| NXP Semiconductors
| Logic Products Group
| IBIS model of NX3DV3899
| DUAL DOUBLE-POLE DOUBLE-THROW ANALOG SWITCH
|[Packages]:
|[Package1]: HXQFN16U (HR) 16-pins package
|[Package2]: XQFN16 (GU) 16-pins Package
[IBIS Ver]   3.2
[File Name]   nx3dv3899.ibs
[File Rev]   1.0
[Date]   17-Jun-2011
[Source]   File created from simulations by LPG
   NXP Semiconductors Nijmegen
[Notes]   V1.0   Ibis model.
   Revision History
   Version Date   Author/ Description
   Editor
   1.0   Juny  2011   RRV   Initial Model
   Remarks: - The Power Clamp curves have been omitted from the input
   since there is no power clamp diode.
   - IBISCHK 5.0.1 used
   - Following notes/warnings are caused by normal switch behaviour:
   'Series_MOSFET has Decreasing Current'
   'Series_MOSFET data is non-monotonic'
[Disclaimer]
   NXP Semiconductors warrants and represents that the IBIS model
   identified herein is owned by NXP Semiconductors (NXP). The
   model provided is not warranted as fully representing all of the
   operating characteristics and specifications of the semiconductor
   products to which the model relates.  Moreover, unless there is a
   signed, written agreement to the contrary, this IBIS model is
   furnished on an "as is" basis without support or warranty of any
   kind, either expressed or implied, regarding the use thereof, and
   NXP specifically disclaims all implied warranties of
   merchantability and fitness of the model for any purpose.
   NXP does not assume any liability arising out of the application
   or use of this IBIS model including infringement of patents and
   copyrights, nor does NXP convey any license under its patents and
   copyrights or the rights of others.
   NXP provides IBIS models as a service to our customers. You and
   your company shall not distribute, convey, sell, or give these models
   to anyone else without receiving prior written permission from
   NXP.
   NXP reserves the right to make changes without notice to these
   IBIS models to improve reliability, function, or design.
   Please be aware that your receipt and subsequent use of the IBIS
   information provided shall serve as acceptance of the terms and
   conditions of this agreement.  If you do not accept these terms,
   you should return or destroy the IBIS models and any other
   accompanying information immediately.
[Copyright]
   (C) Copyright 2011 NXP Semiconductors
   All rights reserved
|   Info for  HXQFN16U (HR) 16-pins package
[Component]   NX3DV3899_HR
[Manufacturer]   NXP Semiconductors
[Package]
|   Typ   Min   Max
R_pkg   6.915E-02   6.329E-02   7.890E-02
L_pkg   1.056E-09   9.663E-10   1.206E-09
C_pkg   1.547E-13   1.500E-13   1.640E-13
[Pin] signal_name   model_name   R_pin   L_pin   C_pin
   1   1Y0   NX3DV3899_TERM1 7.110E-02 1.086E-09 1.548E-13
   2   1S   NX3DV3899_CTRLIN 6.330E-02 9.663E-10 1.500E-13
   3   2Y1   NX3DV3899_TERM1 6.329E-02 9.663E-10 1.502E-13
   4   2Z   NX3DV3899_TERM2 7.110E-02 1.086E-09 1.550E-13
   5   2Y0   NX3DV3899_TERM1 7.889E-02 1.206E-09 1.639E-13
   6   GND   GND 6.330E-02 9.663E-10 1.500E-13
   7   3Y1   NX3DV3899_TERM1 6.330E-02 9.664E-10 1.500E-13
   8   3Z   NX3DV3899_TERM2 7.890E-02 1.206E-09 1.639E-13
   9   3Y0   NX3DV3899_TERM1 7.110E-02 1.086E-09 1.549E-13
   10   2S   NX3DV389_CTRLIN 6.330E-02 9.663E-10 1.500E-13
   11   4Y1   NX3DV3899_TERM1 6.330E-02 9.663E-10 1.500E-13
   12   4Z   NX3DV3899_TERM2 7.110E-02 1.086E-09 1.548E-13
   13   4Y0   NX3DV3899_TERM1 7.890E-02 1.206E-09 1.640E-13
   14   VCC   POWER 6.330E-02 9.663E-10 1.502E-13
   15   1Y1   NX3DV3899_TERM1 6.329E-02 9.663E-10 1.500E-13
   16   1Z   NX3DV3899_TERM2 7.889E-02 1.206E-09 1.638E-13
|   Info for  XQFN16 (GU) 16-pins Package
[Component]   NX3DV3899_GU
[Manufacturer]   NXP Semiconductors
[Package]
|   Typ   Min   Max
R_pkg   5.140E-02   3.890E-02   6.732E-02
L_pkg   6.558E-10   4.951E-10   8.595E-10
C_pkg   1.383E-13   1.222E-13   1.574E-13
[Pin] signal_name   model_name   R_pin   L_pin   C_pin
   1   1Y0   NX3DV3899_TERM1 4.876E-02 6.219E-10 1.378E-13
   2   1S   NX3DV3899_CTRLIN 4.180E-02 5.321E-10 1.297E-13
   3   2Y1   NX3DV3899_TERM1 4.031E-02 5.157E-10 1.286E-13
   4   2Z   NX3DV3899_TERM2 3.890E-02 4.951E-10 1.224E-13
   5   2Y0   NX3DV3899_TERM1 6.525E-02 8.353E-10 1.574E-13
   6   GND   GND 5.937E-02 7.574E-10 1.499E-13
   7   3Y1   NX3DV3899_TERM1 5.708E-02 7.305E-10 1.481E-13
   8   3Z   NX3DV3899_TERM2 5.905E-02 7.534E-10 1.454E-13
   9   3Y0   NX3DV3899_TERM1 5.082E-02 6.479E-10 1.359E-13
   10   2S   NX3DV389_CTRLIN 4.579E-02 5.835E-10 1.301E-13
   11   4Y1   NX3DV3899_TERM1 4.055E-02 5.163E-10 1.241E-13
   12   4Z   NX3DV3899_TERM2 6.732E-02 8.595E-10 1.550E-13
   13   4Y0   NX3DV3899_TERM1 3.894E-02 4.957E-10 1.222E-13
   14   VCC   POWER 4.994E-02 6.366E-10 1.349E-13
   15   1Y1   NX3DV3899_TERM1 5.901E-02 7.529E-10 1.454E-13
   16   1Z   NX3DV3899_TERM2 5.948E-02 7.590E-10 1.459E-13
[Series Pin Mapping]  pin_2  model_name   function_table_group
 4   5   NX3DV3899_SWITCH1   1
 4   3   NX3DV3899_SWITCH1   2
 8   9   NX3DV3899_SWITCH1   1
 8   7   NX3DV3899_SWITCH1   2
12   13   NX3DV3899_SWITCH1   1
12   11   NX3DV3899_SWITCH1   2
16   1   NX3DV3899_SWITCH1   1
16   15   NX3DV3899_SWITCH1   2
 5   4   NX3DV3899_SWITCH2   3
 3   4   NX3DV3899_SWITCH2   4
 9   8   NX3DV3899_SWITCH2   3
 7   8   NX3DV3899_SWITCH2   4
13   12   NX3DV3899_SWITCH2   3
11   12   NX3DV3899_SWITCH2   4
 1   16   NX3DV3899_SWITCH2   3
15   16   NX3DV3899_SWITCH2   4
[Series Switch Groups]
| Function Group States
On 1 /   | Z  to Y0, S=Low
On 2 /   | Z  to Y1, S=High
On 3 /   | Y0 to Z, S=Low
On 4 /   | Y1 to Z, S=High
[Model Selector]   NX3DV3899_SWITCH1
NX3DV3899_SWITCH1_33   3.3V-Vcc Series switch model
NX3DV3899_SWITCH1_25   2.5V-Vcc Series switch model
NX3DV3899_SWITCH1_18   1.8V-Vcc Series switch model
NX3DV3899_SWITCH1_15   1.5V-Vcc Series switch model
[Model Selector]   NX3DV3899_SWITCH2
NX3DV3899_SWITCH2_33   3.3V-Vcc Series switch model
NX3DV3899_SWITCH2_25   2.5V-Vcc Series switch model
NX3DV3899_SWITCH2_18   1.8V-Vcc Series switch model
NX3DV3899_SWITCH2_15   1.5V-Vcc Series switch model
[Model Selector]   NX3DV3899_TERM1
NX3DV3899_TERM1_33   3.3V-Vcc Series switch I/O model
NX3DV3899_TERM1_25   2.5V-Vcc Series switch I/O model
NX3DV3899_TERM1_18   1.8V-Vcc Series switch I/O model
NX3DV3899_TERM1_15   1.5V-Vcc Series switch I/O model
[Model Selector]   NX3DV3899_CTRLIN
NX3L_CTRLIN_33   3.3V-Vcc input model
NX3L_CTRLIN_25   2.5V-Vcc input model
NX3L_CTRLIN_18   1.8V-Vcc input model
NX3L_CTRLIN_15   1.5V-Vcc input model
[Model Selector]   NX3DV3899_TERM2
NX3DV3899_TERM2_33   3.3V-Vcc Series switch I/O model
NX3DV3899_TERM2_25   2.5V-Vcc Series switch I/O model
NX3DV3899_TERM2_18   1.8V-Vcc Series switch I/O model
NX3DV3899_TERM2_15   1.5V-Vcc Series switch I/O model
[Model Selector]   NX3DV389_CTRLIN
NX3L_CTRLIN_33   3.3V-Vcc input model
NX3L_CTRLIN_25   2.5V-Vcc input model
NX3L_CTRLIN_18   1.8V-Vcc input model
NX3L_CTRLIN_15   1.5V-Vcc input model
|   Model NX3DV3899_SWITCH1_33
[Model]   NX3DV3899_SWITCH1_33
Model_type   Series_switch
C_comp   32.2940pF   29.6500pF   35.6150pF
| ON capacitance of switch
|Ambient temperature:   25   85   -40
[Temperature Range]   30   90   -35
[Voltage Range]   3.3   3.0   3.6
[Off]
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[On]
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|   Model NX3DV3899_SWITCH1_25
[Model]   NX3DV3899_SWITCH1_25
Model_type   Series_switch
C_comp   33.4930pF   30.9360pF   36.1910pF
| ON capacitance of switch
|Ambient temperature:   25   85   -40
[Temperature Range]   30   90   -35
[Voltage Range]   2.5   2.3   2.7
[Off]
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[On]
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|   Model NX3DV3899_SWITCH1_18
[Model]   NX3DV3899_SWITCH1_18
Model_type   Series_switch
C_comp   33.7050pF   31.2860pF   36.3240pF
| ON capacitance of switch
|Ambient temperature:   25   85   -40
[Temperature Range]   30   90   -35
[Voltage Range]   1.8   1.65   1.95
[Off]
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[On]
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|   Model NX3DV3899_SWITCH1_15
[Model]   NX3DV3899_SWITCH1_15
Model_type   Series_switch
C_comp   31.1850pF   27.5650pF   35.7310pF
| ON capacitance of switch
|Ambient temperature:   25   85   -40
[Temperature Range]   30   90   -35
[Voltage Range]   1.5   1.4   1.6
[Off]
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[On]
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|   Model NX3DV3899_SWITCH2_33
[Model]   NX3DV3899_SWITCH2_33
Model_type   Series_switch
C_comp   32.2960pF   29.7210pF   35.6190pF
| ON capacitance of switch
|Ambient temperature:   25   85   -40
[Temperature Range]   30   90   -35
[Voltage Range]   3.3   3.0   3.6
[Off]
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[On]
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|   Model NX3DV3899_SWITCH2_25
[Model]   NX3DV3899_SWITCH2_25
Model_type   Series_switch
C_comp   33.4875pF   30.9420pF   36.1700pF
| ON capacitance of switch
|Ambient temperature:   25   85   -40
[Temperature Range]   30   90   -35
[Voltage Range]   2.5   2.3   2.7
[Off]
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[On]
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|   Model NX3DV3899_SWITCH2_18
[Model]   NX3DV3899_SWITCH2_18
Model_type   Series_switch
C_comp   33.7090pF   31.3130pF   36.3320pF
| ON capacitance of switch
|Ambient temperature:   25   85   -40
[Temperature Range]   30   90   -35
[Voltage Range]   1.8   1.65   1.95
[Off]
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[On]
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|   Model NX3DV3899_SWITCH2_15
[Model]   NX3DV3899_SWITCH2_15
Model_type   Series_switch
C_comp   31.1580pF   27.0770pF   35.8290pF
| ON capacitance of switch
|Ambient temperature:   25   85   -40
[Temperature Range]   30   90   -35
[Voltage Range]   1.5   1.4   1.6
[Off]
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[On]
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| Models and submodels in the file (20): NX3DV3899_TERM1_33 (Terminator), NX3DV3899_SWITCH1_33 (Series_switch), NX3DV3899_TERM1_25 (Terminator), NX3DV3899_SWITCH1_25 (Series_switch), NX3DV3899_TERM1_18 (Terminator), NX3DV3899_SWITCH1_18 (Series_switch), NX3DV3899_TERM1_15 (Terminator), NX3DV3899_SWITCH1_15 (Series_switch), NX3L_CTRLIN_33 (Input), NX3L_CTRLIN_25 (Input), NX3L_CTRLIN_18 (Input), NX3L_CTRLIN_15 (Input), NX3DV3899_TERM2_33 (Terminator), NX3DV3899_SWITCH2_33 (Series_switch), NX3DV3899_TERM2_25 (Terminator), NX3DV3899_SWITCH2_25 (Series_switch), NX3DV3899_TERM2_18 (Terminator), NX3DV3899_SWITCH2_18 (Series_switch), NX3DV3899_TERM2_15 (Terminator), NX3DV3899_SWITCH2_15 (Series_switch)
